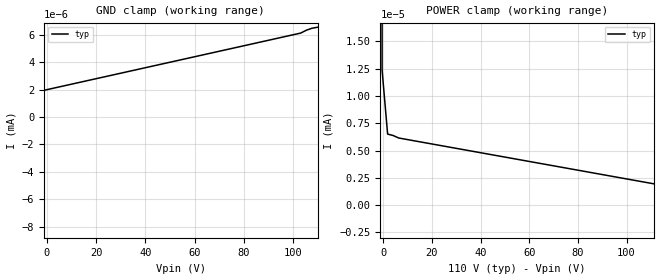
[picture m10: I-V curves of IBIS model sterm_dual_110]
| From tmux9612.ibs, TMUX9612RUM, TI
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| sterm_dual_110
[Model]   sterm_dual_110
Model_type   Terminator
|   typ   min   max
C_comp   6.362683e-12   NA   NA
[Voltage Range]   110   NA   NA
[Temperature Range]   27   NA   NA
[Power Clamp Reference]   110   NA   NA
[GND Clamp Reference]   0   NA   NA
[GND Clamp]
|   Voltage   I(typ)   I(min)   I(max)
-115V     -2.415A    NA         NA
-110.5V   -102.8nA   NA         NA
-108.2V   -2.339nA   NA         NA
103.2V    6.135nA    NA         NA
107.7V    6.485nA    NA         NA
110V      6.559nA    NA         NA
[POWER Clamp]
|   Voltage   I(typ)   I(min)   I(max)
-5V       1.055A     NA         NA
-2.727V   432.7mA    NA         NA
-455mV    12.37nA    NA         NA
1.818V    6.511nA    NA         NA
6.364V    6.153nA    NA         NA
220V      -2.413nA   NA         NA
